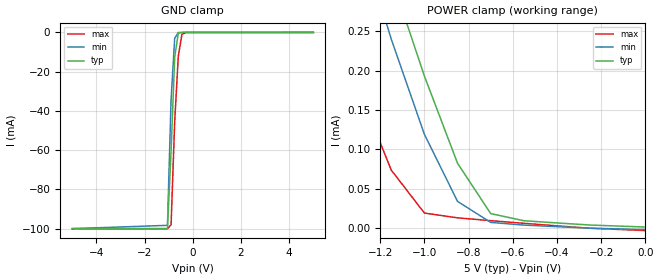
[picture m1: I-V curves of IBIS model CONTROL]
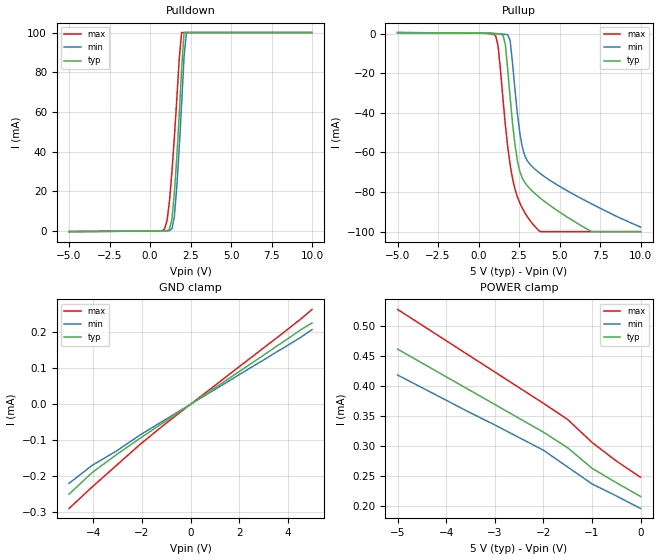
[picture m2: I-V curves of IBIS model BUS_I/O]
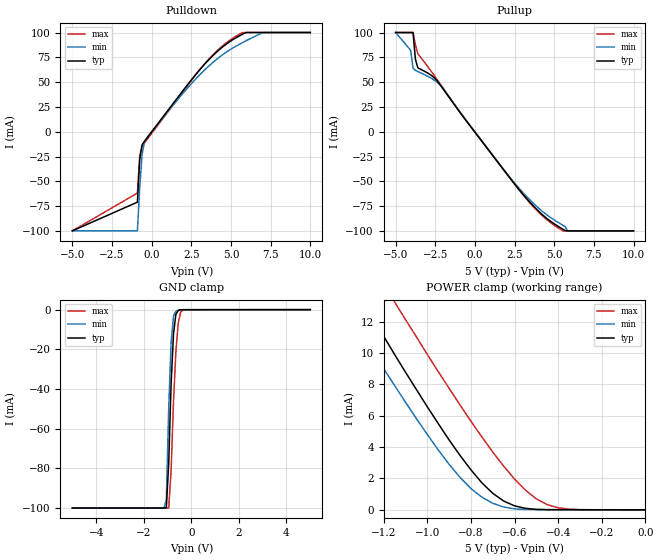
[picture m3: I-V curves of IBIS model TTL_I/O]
|   Texas Instruments Incorporated
|   Data Transmissions Products
|   IBIS Model for SN75976A
|   56DGG Package
[IBIS Ver]   2.1
[Comment char]   |_char
[File name]   75976a.ibs
[File Rev]   2.0
[Date]   8Oct97
[Source]   File originated at Texas Instruments Incorporated.
   Data Transmission Products Group. All data based on
   Bench Measurements.
[Notes]   File created by Thomas Fisher
[Disclaimer]
(C) Copyright Texas Instruments Incorporated 1997
   All rights reserved
  Texas Instruments Incorporated hereby grants the user of this IBIS
model a non-exclusive, nontransferable license to use this IBIS model
under the following terms.  Before using this IBIS model, the user
should read this license.  If the user does not accept these terms,
the IBIS model should be returned to Texas Instruments within 30 days.
  The user is granted this license only to use the IBIS model and
is not granted rights to sell, load, rent, lease or license the IBIS
model in whole or in part, or in modified form to anyone other than
user.  User may modify the IBIS model to suit its specific applications
but rights to derivative works and such modifications shall belong to
Texas Instruments.
  This IBIS model is provided on an "AS IS" basis and Texas Instruments
makes absolutely no warranty with respect to the information contained
herein.  TEXAS INSTRUMENTS DISCLAIMS AND CUSTOMER WAIVES ALL WARRANTIES,
EXPRESS OR IMPLIED, INCLUDING WARRANTIES OF MERCHANTABILITY OR FITNESS
FOR A PARTICULAR PURPOSE. The entire risk as to quality and performance
is with the Customer. ACCORDINGLY, IN NO EVENT SHALL THE COMPANY BE LIABLE
FOR ANY DAMAGES, WHETHER IN CONTRACT OR TORT,INCLUDING ANY LOST PROFITS
OR OTHER INCIDENTAL, CONSEQUENTIAL, EXEMPLARY, OR PUNITIVE DAMAGES ARISING
OUT OF THE USE OR APPLICATION OF THE IBIS model provided in this package.
Further, Texas Instruments reserves the right to discontinue or make changes
without notice to any product herein to improve reliability, function, or
design. Texas Instruments does not convey any license under patent rights
or any other intellectual property rights, including those of third parties.
Contact Texas Instruments at ATTN:DATA TRANSMISSIONS
Thomas Fisher  8505 Forest Lane, M/S 8710, Dallas, TX 75243-4136
[Copyright]   Copyright 1997, Texas Instruments, All Rights Reserved
[Component]   SN75976ADGG
[Manufacturer]  Texas Instruments Incorporated
[Package]
|   typ   min   max
R_pkg   0.032   0.024   0.041
L_pkg   4.018nH   2.746nH   6.620nH
C_pkg   0.461pF   0.261pF   0.854pF
[Pin]   signal_name   model_name   R_pin   L_pin   C_pin
1   GND   GND   0.038   6.533n   0.795p
2   BSR   CONTROL   0.038   5.957n   0.824p
3   CRE   CONTROL   0.039   5.485n   0.725p
4   1A   TTL_I/O   0.040   5.037n   0.634p
5   1DE/RE   CONTROL   0.040   4.575n   0.508p
6   2A   TTL_I/O   0.039   4.053n   0.408p
7   2DE/RE   CONTROL   0.031   3.473n   0.357p
8   3A   TTL_I/O   0.028   3.292n   0.367p
9   3DE/RE   CONTROL   0.027   3.275n   0.353p
10   4A   TTL_I/O   0.027   3.090n   0.318p
11   4DE/RE   CONTROL   0.027   2.879n   0.277p
12   VCC   POWER   0.027   2.826n   0.286p
13   GND   GND   0.028   2.866n   0.289p
14   GND   GND   0.028   2.793n   0.288p
15   GND   GND   0.028   2.799n   0.288p
16   GND   GND   0.026   2.802n   0.288p
17   GND   GND   0.025   2.746n   0.282p
18   VCC   POWER   0.026   2.838n   0.284p
19   5A   TTL_I/O   0.025   2.952n   0.310p
20   5DE/RE   CONTROL   0.026   3.272n   0.328p
21   6A   TTL_I/O   0.028   3.293n   0.373p
22   6DE/RE   CONTROL   0.031   3.478n   0.318p
23   7A   TTL_I/O   0.039   4.108n   0.359p
24   7DE/RE   CONTROL   0.040   4.592n   0.524p
25   8A   TTL_I/O   0.040   5.061n   0.652p
26   8DE/RE   CONTROL   0.038   5.507n   0.747p
27   9A   TTL_I/O   0.038   6.003n   0.848p
28   9DE/RE   CONTROL   0.036   6.519n   0.769p
29   1B-   BUS_I/O   0.036   6.531n   0.769p
30   1B+   BUS_I/O   0.038   5.994n   0.847p
31   2B-   BUS_I/O   0.038   5.511n   0.747p
32   2B+   BUS_I/O   0.040   5.067n   0.653p
33   3B-   BUS_I/O   0.040   4.606n   0.525p
34   3B+   BUS_I/O   0.040   4.110n   0.423p
35   4B-   BUS_I/O   0.030   3.477n   0.366p
36   4B+   BUS_I/O   0.026   3.289n   0.323p
37   5B-   BUS_I/O   0.025   2.848n   0.261p
38   5B+   BUS_I/O   0.024   2.943n   0.312p
39   VCC   POWER   0.026   2.841n   0.285p
40   GND   GND   0.026   2.773n   0.284p
41   GND   GND   0.027   2.834n   0.289p
42   GND   GND   0.028   2.803n   0.287p
43   GND   GND   0.028   2.817n   0.288p
44   GND   GND   0.027   2.836n   0.291p
45   VCC   POWER   0.027   2.824n   0.287p
46   6B-   BUS_I/O   0.027   3.242n   0.375p
47   6B+   BUS_I/O   0.027   3.000n   0.312p
48   7B-   BUS_I/O   0.027   3.298n   0.330p
49   7B+   BUS_I/O   0.029   3.305n   0.375p
50   8B-   BUS_I/O   0.031   3.858n   0.441p
51   8B+   BUS_I/O   0.040   4.131n   0.397p
52   9B-   BUS_I/O   0.041   4.664n   0.481p
53   9B+   BUS_I/O   0.040   5.089n   0.654p
54   CDE0   CONTROL   0.040   5.566n   0.753p
55   CDE1   CONTROL   0.038   6.009n   0.854p
56   CDE2   CONTROL   0.039   6.620n   0.810p
[Diff_pin]   inv_pin   vdiff   tdelay_typ   tdelay_min   tdelay_max
| The 'XB+' pin is diff_pin and the 'XB-' pin is the inv_pin
30   29   200mV   0 0 0
32   31   200mV   0 0 0
34   33   200mV   0 0 0
36   35   200mV   0 0 0
38   37   200mV   0 0 0
47   46   200mV   0 0 0
49   48   200mV   0 0 0
51   50   200mV   0 0 0
53   52   200mV   0 0 0
| Models and submodels in the file (3): CONTROL (Input), BUS_I/O (I/O), TTL_I/O (I/O)
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|   Control Inputs  Model
[Model]   CONTROL
Model_type   Input
|Signals   CDE0,CDE1,CDE2,CRE,BSR,1DE/RE,2DE/RE,3DE/RE,4DE/RE,5DE/RE,
|   6DE/RE,7DE/RE,8DE/RE,9DE/RE
Vinh = 2.0
Vinl = 0.8
|   typ   min   max
C_comp   1.0pF   NA   NA
|   typ   min   max
[Temperature Range]   25.0   0.0   115.0
[Voltage range]   5.00V   4.75V   5.25V
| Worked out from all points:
|   GND clamp passes 1 mA (typ) near -0.61 V on its own axis
|   POWER clamp passes 1 mA (typ) near -1.89 V on its own axis
[Power_clamp]
| Note that the[POWER_clamp]voltage table is referenced to Vcc
| and is calculated using Vtable=Vcc - Vmeasured.
|   Voltage   I(typ)   I(min)   I(max)
-5V       100.1mA    100.1mA    100.1mA
-1.45V    589uA      524uA      297uA
-1.3V     452uA      378uA      178uA
-1.15V    319uA      240uA      73.6uA
-1V       193uA      119uA      19uA
-850mV    82.2uA     33.8uA     12.9uA
-700mV    18.3uA     7.1uA      9.32uA
-550mV    9.25uA     3.69uA     5.96uA
-250mV    3.77uA     -236nA     -316nA
0V        1.23uA     -2.05uA    -3.26uA
[GND_clamp]
|   Voltage   I(typ)   I(min)   I(max)
-5V       -99.96mA   -99.95mA   -99.96mA
-1.05V    -99.96mA   -98.27mA   -99.96mA
-900mV    -60.47mA   -34.25mA   -97.98mA
-750mV    -12.56mA   -2.99mA    -45.43mA
-600mV    -430uA     -50.9uA    -12.05mA
-450mV    -32uA      -39.7uA    -1.04mA
-300mV    -30uA      -39.6uA    -45.7uA
5V        -1.2uA     -6.07uA    -3.82uA
|   Bus Input/Output  Model
[Model]   BUS_I/O
Model_type   I/O
|Signals   1B-,1B+,2B-,2B+,3B-,3B+,4B-,4B+,5B-,5B+,6B-,6B+,7B-,7B+,
|   8B-,8B+,9B-,9B+
Cref = 15pf
|Rref = parallel network - see datasheet  (Figure 1) for configuration
Vinh = 3.0
Vinl = 1.0
|   typ   min   max
C_comp   1.0pF   NA   NA
|   typ   min   max
[Temperature Range]   25.0   0.0   115.0
[Voltage range]   5.0V   4.75V   5.25V
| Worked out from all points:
|   slope of the pulldown table from 0 to 0.75 V, typ, clamps not added: 10.1 kohm
|   slope of the pullup table from 0 to 0.75 V, typ, clamps not added: 6.25 kohm
[Pulldown]
|   Voltage   I(typ)   I(min)   I(max)
-5V       -250uA     -230uA     -290uA
900mV     100uA      89.5uA     1.108mA
1.05V     168uA      115uA      5.315mA
1.2V      943uA      201uA      15.16mA
1.35V     6.059mA    1.056mA    29.72mA
1.5V      18.95mA    7.333mA    47.16mA
1.65V     37.08mA    22.18mA    66.24mA
1.8V      58.46mA    41.79mA    86.41mA
1.95V     81.68mA    64.09mA    100.1mA
2.1V      100.1mA    88.1mA     100.1mA
2.25V     100.1mA    100mA      100.1mA
10V       100.1mA    100.1mA    100.1mA
[Pullup]
|   Voltage   I(typ)   I(min)   I(max)
| Note that the[Pullup]voltage table is referenced to Vcc
| and is calculated using Vtable=Vcc - Vmeasured.
-5V       495uA      473uA      547uA
1.05V     -100uA     99.4uA     -960uA
1.2V      -220uA     -9.24uA    -6mA
1.5V      -680uA     -240uA     -32.23mA
1.8V      -17.98mA   -550uA     -57.09mA
1.95V     -32.23mA   -3.58mA    -66.15mA
2.4V      -64.27mA   -40.59mA   -82.49mA
2.7V      -72.93mA   -57.25mA   -88.08mA
3V        -76.69mA   -64.03mA   -92.29mA
3.75V     -82.62mA   -70.24mA   -99.68mA
6.9V      -99.66mA   -85.6mA    -99.96mA
10V       -99.96mA   -97.74mA   -99.96mA
[Power_clamp]
| Note that the[POWER_clamp]voltage table is referenced to Vcc
| and is calculated using Vtable=Vcc - Vmeasured.
|   Voltage   I(typ)   I(min)   I(max)
-5V       461uA      418uA      527uA
-4.5V     438uA      397uA      501uA
-4V       415uA      376uA      475uA
-3.5V     392uA      355uA      449uA
-3V       369uA      335uA      423uA
-2.5V     346uA      314uA      397uA
-2V       323uA      293uA      371uA
-1.5V     297uA      265uA      344uA
-1V       263uA      237uA      306uA
-500mV    239uA      217uA      275uA
0V        216uA      196uA      248uA
[GND_clamp]
|   Voltage   I(typ)   I(min)   I(max)
-5V       -250uA     -220uA     -290uA
-4.05V    -190uA     -170uA     -230uA
-3.05V    -140uA     -130uA     -170uA
-2.05V    -93.4uA    -84.2uA    -110uA
-1.05V    -47.8uA    -43.1uA    -55uA
3.95V     180uA      162uA      206uA
4.55V     208uA      187uA      238uA
5V        226uA      208uA      264uA
[Ramp]
| Note: Ramp rate measured on single-ended Driver Output.
|   typ   min   max
dV/dt_r   1.504/5.704ns   1.536/5.024ns   1.600/6.560ns
dV/dt_f   1.504/2.056ns   1.536/1.896ns   2.048/2.808ns
R_load = 205ohm | Note: These are single ended driver measurements
|   with 205ohm line-to-line termination and 15.0pF
|   line-to-ground capacitive load
|   TTL Input/Output  Model
[Model]   TTL_I/O
Model_type   I/O
| Signals   1A,2A,3A,4A,5A,6A,7A,8A,9A
Vinh = 2.0
Vinl = 0.8
| variable   typ   min   max
C_comp   1.0pF   NA   NA
|   typ   min   max
[Temperature Range]   25.0   0.0   115.0
[Voltage range]   5.0V   4.75V   5.25V
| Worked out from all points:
|   slope of the pulldown table from 0 to 0.75 V, typ, clamps not added: 47.5 ohm
|   slope of the pullup table from 0 to 0.75 V, typ, clamps not added: 47.8 ohm
|   GND clamp passes 1 mA (typ) near -0.58 V on its own axis
|   POWER clamp passes 1 mA (typ) near -0.69 V on its own axis
[Pulldown]
|   Voltage   I(typ)   I(min)   I(max)
-5V       -99.96mA   -99.96mA   -99.96mA
-900mV    -71.03mA   -99.96mA   -61.9mA
-750mV    -27.19mA   -55.81mA   -23.8mA
-600mV    -13.17mA   -22.43mA   -14.46mA
-450mV    -9.55mA    -10.13mA   -11.18mA
2.55V     53.24mA    49.24mA    52.62mA
3.6V      72.63mA    66.21mA    73.03mA
4.5V      85.85mA    77.96mA    86.96mA
5.7V      98.11mA    89.65mA    99.83mA
6V        100.1mA    92.17mA    100.1mA
7.05V     100.1mA    100.1mA    100.1mA
10V       100.1mA    100.1mA    100.1mA
[Pullup]
|   Voltage   I(typ)   I(min)   I(max)
| Note that the[Pullup]voltage table is referenced to Vcc
| and is calculated using Vtable=Vcc - Vmeasured.
-5V       100.1mA    100.1mA    100.1mA
-4.05V    100.1mA    82.14mA    100.1mA
-3.9V     100.1mA    64.04mA    100.1mA
-3.75V    73.12mA    61.82mA    87.55mA
-3.6V     64.47mA    60.72mA    78.63mA
-2.7V     56.26mA    53.44mA    59.73mA
-2.1V     45.3mA     45.43mA    46.14mA
2.25V     -47.55mA   -46.9mA    -47.65mA
4.5V      -86.99mA   -83.44mA   -88.21mA
5.55V     -98.33mA   -94.32mA   -99.94mA
5.85V     -99.96mA   -99.97mA   -99.96mA
10V       -99.96mA   -99.97mA   -99.96mA
[GND_clamp]
|   Voltage   I(typ)   I(min)   I(max)
| Outputs in Tri-state.
-5V       -99.96mA   -99.96mA   -99.96mA
-1.15V    -99.96mA   -99.96mA   -99.96mA
-1.05V    -99.96mA   -95.87mA   -99.96mA
-950mV    -77.26mA   -49.46mA   -99.96mA
-850mV    -37.66mA   -16.92mA   -81.31mA
-750mV    -12.4mA    -3.23mA    -46.67mA
-650mV    -2.39mA    -870uA     -21.25mA
-550mV    -470uA     -210uA     -6.75mA
-450mV    -80uA      -47uA      -1.32mA
-350mV    -34uA      -40uA      -160uA
5V        -3.6uA     -4.3uA     -2.6uA
[POWER_clamp]
|   Voltage   I(typ)   I(min)   I(max)
| Note that the [POWER_clamp] voltage table is referenced to Vcc
| and is calculated using Vtable = Vcc - Vmeasured.
| Outputs in Tri-state.
-5V       100.1mA    100.1mA    100.1mA
-1.4V     15.71mA    13.44mA    18.92mA
-1.3V     13.37mA    11.21mA    16.65mA
-1.25V    12.22mA    10.1mA     15.5mA
-1.15V    9.901mA    7.923mA    13.25mA
-1.1V     8.771mA    6.86mA     12.13mA
-850mV    3.468mA    2.072mA    6.682mA
-750mV    1.723mA    808uA      4.65mA
-650mV    561uA      177uA      2.787mA
-550mV    93.7uA     21.2uA     1.253mA
-450mV    12.2uA     9.55uA     329uA
0V        -320nA     -336nA     -244nA
[Ramp]
|   typ   min   max
dV/dt_r   4.192/1.320ns   4.384/1.220ns   3.904/1.408ns
dV/dt_f   4.192/1.396ns   3.936/1.248ns   4.320/1.464ns
R_load = 1MOhm   | note Represents an open
